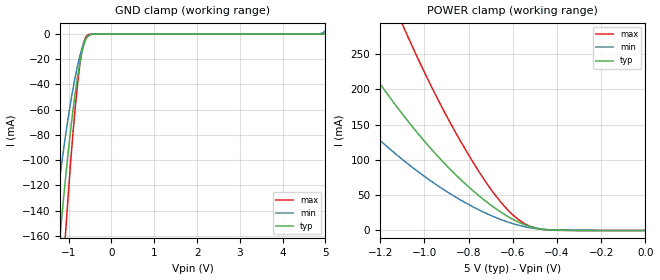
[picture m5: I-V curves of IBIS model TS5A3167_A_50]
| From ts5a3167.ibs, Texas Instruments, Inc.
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[Model]   TS5A3167_A_50
Model_type  Terminator
| variable   typ   min   max
C_comp   18.19pF   16.22pF   19.57pF
| C_tri-state   18.19pF   16.22pF   19.57pF
[Temperature Range]   40   100   -40
| Ambient temperature   25   85   -40
[Voltage range]   5   4.5   5.5
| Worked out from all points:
|   GND clamp passes 1 mA (typ) near -0.52 V on its own axis
|   POWER clamp passes 1 mA (typ) near -0.43 V on its own axis
[GND Clamp]
| TS5A3167_A_50
|   Voltage   I(typ)   I(min)   I(max)
-5V       -2.49A     -1.885A    -3.22A
-1.395V   -239.8mA   -167.3mA   -341.2mA
-1.35V    -220.4mA   -153.8mA   -313.3mA
-1.185V   -154.1mA   -107.9mA   -216.8mA
-1.07V    -112.8mA   -79.45mA   -156mA
-905mV    -61.93mA   -44.43mA   -80.7mA
-775mV    -30.06mA   -22.42mA   -34.21mA
-725mV    -20.27mA   -15.62mA   -20.78mA
-660mV    -10.28mA   -8.518mA   -8.393mA
-540mV    -1.353mA   -1.472mA   -499uA
4.78V     228.6pA    26.8uA     89.79pA
5V        1.593nA    2.789mA    96.81pA
[POWER Clamp]
| TS5A3167_A_50
|   Voltage   I(typ)   I(min)   I(max)
-5V       3.28A      2.411A     4.661A
-1.66V    447mA      282.6mA    762.7mA
-1.365V   285.6mA    177.2mA    498.6mA
-1.1V     165.2mA    100.8mA    292.5mA
-1.075V   155.2mA    94.49mA    274.9mA
-915mV    96.99mA    58.4mA     171.4mA
-780mV    56.3mA     33.49mA    96.83mA
-680mV    31.57mA    18.71mA    50.29mA
-575mV    11.89mA    7.484mA    15.55mA
-525mV    5.882mA    4.033mA    6.372mA
-460mV    1.744mA    1.414mA    1.305mA
-84.45fV  1.593nA    9.498nA    134.1pA
